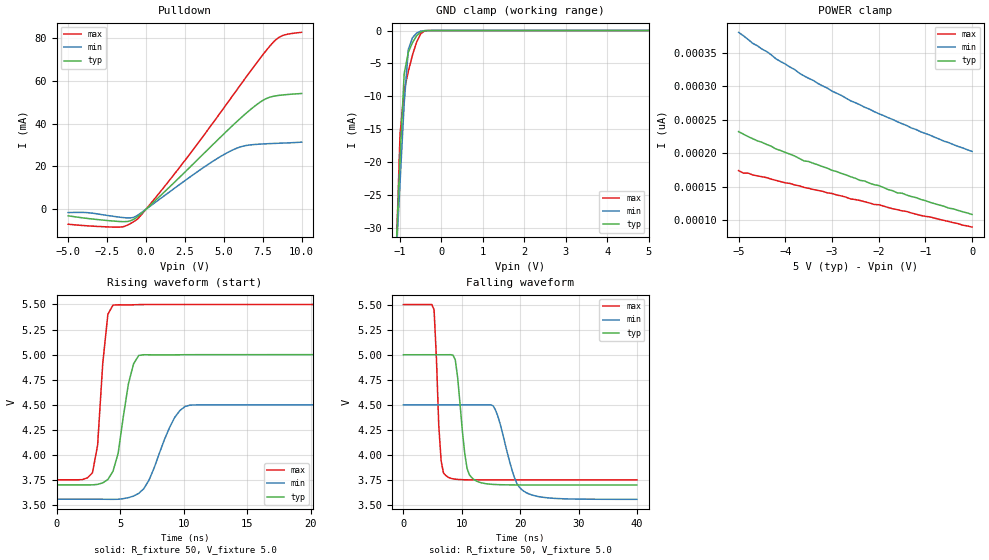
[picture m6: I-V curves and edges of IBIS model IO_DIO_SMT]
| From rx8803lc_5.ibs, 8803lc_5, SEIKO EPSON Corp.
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[Model]   IO_DIO_SMT
Model_type I/O_open_drain
Enable Active-High
Polarity Non-Inverting
Vinh=4.0
Vinl=1.0
C_comp   5p   4p   6p
[Temperature Range] 25   85   -40
[Voltage Range]   5.0   4.5   5.5
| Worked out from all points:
|   slope of the pulldown table from 0 to 0.75 V, typ, clamps not added: 147 ohm
|   GND clamp passes 1 mA (typ) near -0.62 V on its own axis
|   falling waveform, R_fixture 50, V_fixture 5.0: 20-80 % time 1.31ns typ, 2.65ns min, 778ps max; typ from 5 V to 3.7 V
|   rising waveform, R_fixture 50, V_fixture 5.0: 20-80 % time 995ps typ, 1.78ns min, 597ps max; typ from 3.7 V to 5 V
[Pulldown]
-5V       -3.113mA   -1.575mA   -7.017mA
-3.8V     -4.284mA   -1.586mA   -7.76mA
-1.7V     -5.749mA   -3.719mA   -8.376mA
-1.1V     -5.625mA   -4.081mA   -7.102mA
-600mV    -3.875mA   -3.12mA    -4.891mA
2.1V      14.53mA    11.24mA    19.04mA
4.2V      29.54mA    21.97mA    39.38mA
5.6V      39.39mA    27.82mA    53.43mA
7.3V      49.92mA    30.44mA    70.31mA
8.3V      52.98mA    30.79mA    79mA
8.9V      53.53mA    30.96mA    81.52mA
10V       54.13mA    31.37mA    82.75mA
[GND Clamp]
-5V       -674.1mA   -554.3mA   -855.6mA
-1.1V     -34.38mA   -35.36mA   -35.33mA
-1V       -19.42mA   -23.16mA   -15.8mA
-900mV    -6.562mA   -11.13mA   -9.129mA
-800mV    -3.309mA   -2.897mA   -6.201mA
-700mV    -1.841mA   -1.087mA   -3.742mA
-600mV    -807.8uA   -397.8uA   -1.764mA
-500mV    -207.4uA   -91.02uA   -476.4uA
-400mV    -22.76uA   -11uA      -42.64uA
-300mV    -1.222uA   -843.3nA   -1.241uA
5V        108.2pA    215.6pA    81.17pA
[POWER Clamp]
-5V       231.9pA    380.2pA    173.7pA
-4.9V     228.3pA    375.2pA    170.1pA
-4.8V     224.6pA    369.7pA    170.1pA
-4.7V     221.5pA    363.8pA    167.3pA
-3.7V     191.9pA    319.2pA    151pA
-3.6V     188.3pA    315.1pA    148.7pA
-2.6V     164.6pA    277.9pA    131.4pA
-2V       151.4pA    258.8pA    122.8pA
-1.6V     140.5pA    246.7pA    115.5pA
-1.5V     140.1pA    243.7pA    113.7pA
-1.3V     135.1pA    237.4pA    110.5pA
0V        108.2pA    202.4pA    89.36pA
[Falling Waveform]
R_fixture=50
V_fixture=5.0
V_fixture_min=4.5
V_fixture_max=5.5
0s        5V         4.5V       5.5V
5.253ns   5V         4.5V       5.45V
6.465ns   5V         4.5V       3.941V
7.677ns   5V         4.5V       3.778V
8.889ns   4.949V     4.5V       3.759V
10.91ns   3.866V     4.5V       3.753V
12.12ns   3.754V     4.5V       3.753V
15.35ns   3.707V     4.492V     3.753V
21.01ns   3.702V     3.626V     3.752V
40ns      3.702V     3.559V     3.752V
[Rising Waveform]
R_fixture=50
V_fixture=5.0
V_fixture_min=4.5
V_fixture_max=5.5
0s        3.702V     3.559V     3.752V
2.828ns   3.702V     3.559V     3.822V
3.232ns   3.707V     3.559V     4.098V
3.636ns   3.722V     3.558V     4.913V
4.04ns    3.755V     3.558V     5.404V
4.444ns   3.838V     3.558V     5.494V
5.657ns   4.71V      3.574V     5.497V
6.465ns   4.992V     3.617V     5.499V
10.51ns   5V         4.497V     5.5V
40ns      5V         4.5V       5.5V
[Ramp]
R_load=50
dV/dt_r   7.790E-1/9.280E-10   5.649E-1/1.764E-9   1.049E+0/5.440E-10
dV/dt_f   7.788E-1/1.269E-9   5.648E-1/2.654E-9   1.049E+0/6.560E-10
|[End   IO_DIO_SMT
